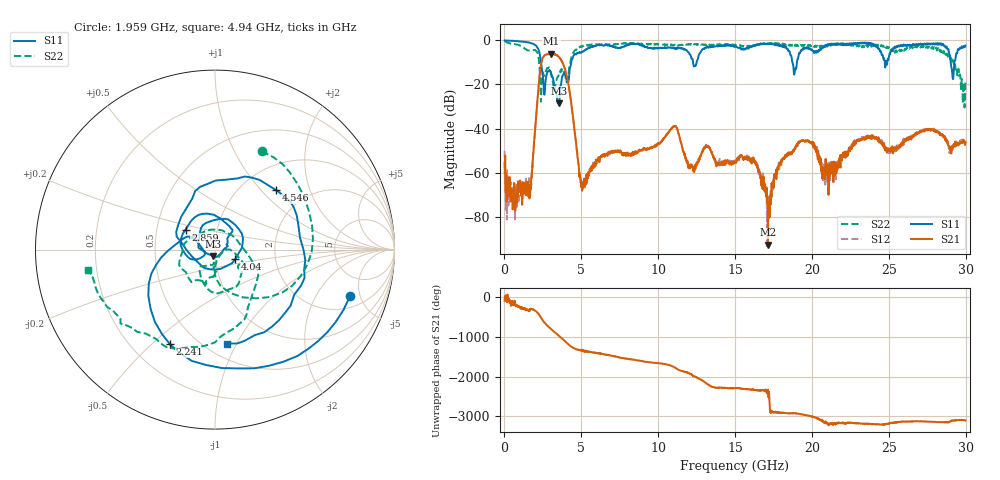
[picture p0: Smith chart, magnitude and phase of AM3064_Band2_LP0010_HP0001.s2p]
# Hz S DB R 50.0
!freq dBS11 angS11 dBS21 angS21 dBS12 angS12 dBS22 angS22
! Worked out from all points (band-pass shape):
!   1600 points, 10 MHz to 29.98 GHz, reference 50 ohm
!   highest |S21| = -6.00 dB at 3.046 GHz (marker M1); lowest = -92.8 dB at 17.14 GHz (marker M2)
!   |S21| within 3 dB of the highest: 2.438 GHz to 3.699 GHz (1.26 GHz wide, 41.1 % of centre)
!   lowest |S11| = -28.6 dB at 3.553 GHz (marker M3), VSWR 1.08, Z = 48.8 - j3.49 ohm
!   |S11| at or under -10 dB: 2.383 GHz to 4.343 GHz (1.959 GHz wide, 58.3 % of centre); 12.27 GHz to 12.5 GHz (229.1 MHz wide, 1.85 % of centre); 18.73 GHz to 19.02 GHz (290.7 MHz wide, 1.54 % of centre)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
!   |S22| runs from -30.5 to -0.2 dB; largest |S21 - S12| = 0.02
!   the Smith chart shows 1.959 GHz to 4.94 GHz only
!   S11 on the Smith chart (normalised r, x): 1.959 GHz: 2.86, -4.03; 2.241 GHz: 0.36, -0.57; 2.859 GHz: 0.70, +0.16; 4.04 GHz: 1.25, -0.13; 4.546 GHz: 1.43, +1.22; 4.94 GHz: 0.63, -0.92
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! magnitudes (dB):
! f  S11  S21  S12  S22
! 10 MHz  0.0  -55.8  -50.1  -0.2
! 1.566 GHz  -0.9  -67.6  -63.9  -4.6
! 1.959 GHz  -2.0  -43.8  -43.5  -4.3
! 2.241 GHz  -4.7  -19.2  -19.2  -9.0
! 2.859 GHz  -14.0  -6.2  -6.2  -12.4
! 3.046 GHz  -15.1  -6.0  -6.0  -15.8
! 3.553 GHz  -28.6  -7.7  -7.6  -14.8
! 4.04 GHz  -18.0  -15.7  -15.7  -18.9
! 4.546 GHz  -6.4  -40.0  -40.0  -4.8
! 4.94 GHz  -5.6  -63.2  -62.1  -2.9
! 5.015 GHz  -5.4  -65.0  -66.2  -3.0
! 10 GHz  -3.5  -47.1  -46.7  -1.8
! 15 GHz  -2.5  -54.9  -55.6  -1.9
! 16.34 GHz  -2.3  -56.2  -54.8  -2.2
! 17.14 GHz  -1.5  -92.8  -84.7  -1.3
! 18.19 GHz  -2.4  -53.6  -53.8  -1.9
! 19.99 GHz  -4.2  -47.0  -46.3  -2.1
! 20.83 GHz  -2.9  -59.2  -57.7  -2.3
! 25 GHz  -8.0  -50.2  -48.6  -3.0
! 28.56 GHz  -2.2  -43.9  -43.2  -4.8
! 29.18 GHz  -17.6  -48.6  -48.0  -8.9
! 29.98 GHz  -2.3  -46.2  -46.6  -19.1
